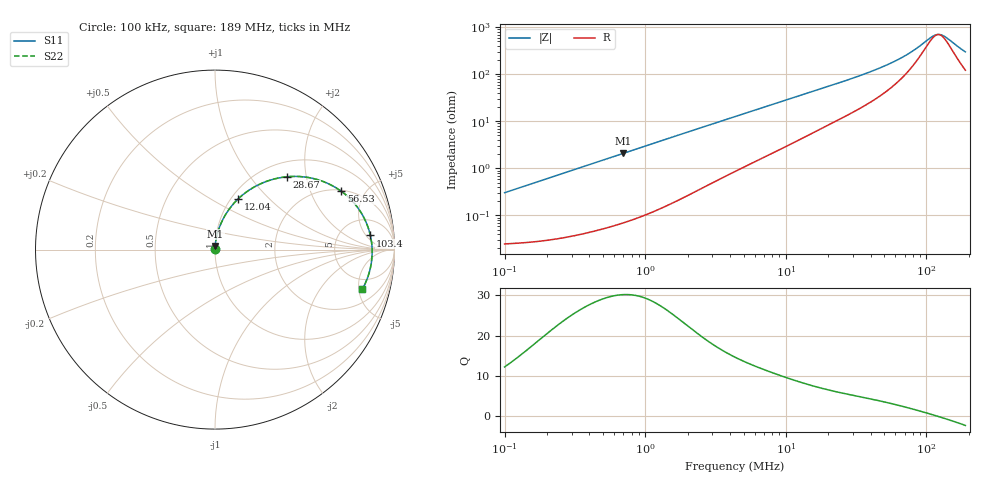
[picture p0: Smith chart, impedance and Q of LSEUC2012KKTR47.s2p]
! LSEUC2012KKTR47  S-PARAMETER MODEL  ( General Type )
! Model Generated by TAIYO YUDEN Corporation (http://www.ty-top.com)
! Version 1.0
! TAIYO YUDEN Control No. 211126
! Copyright(c) 2021 TAIYO YUDEN CO.,LTD. All Rights Reserved.
! Product Description (link to TY-COMPAS)
! https://ds.yuden.co.jp/TYCOMPAS/or/detail?pn=LSEUC2012KKTR47M&u=M
! Products Name : Inductors
! Characteristics :
!  Inductance : 0.47 uH , SRF(min) : -Hz , DC Resistance(max) : 0.027 Ohm
!  Rated Current : Saturation :5000 mA , Temp Rise : 4300 mA (40 degC)
!  Case Size : 2.0 x 1.2 / 0.079 x 0.047 [mm/inch] , Thickness : 1 / 0.039 [mm/inch]
!  (Conditions: Temperature = 25 degC , DC Bias Current/Voltage = 0A / 0V)
! External Node Assignments :
!  1  o---GGG---o  2
! GND o---------o GND
! Frequency Range : 0.1MHz  -  189.042664MHz  [ 402 STEP ]
# MHz S RI R 50
! Freq[MHz].  S11 Real  S11 Imag  S21 Real  S21 Imag  S12 Real  S12 Imag  S22 Real  S22 Imag
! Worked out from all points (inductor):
!   401 points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, 100 kHz to 189 MHz, reference 50 ohm
!   read as one part in series: L = 482 nH near 103.8 kHz
!   highest Q = 30.1 at 697.8 kHz (marker M1), where L = 476 nH
!   self-resonance near 121 MHz
!   S11 on the Smith chart (normalised r, x): 100 kHz: 1.00, +0.01; 12.04 MHz: 1.08, +0.67; 28.67 MHz: 1.29, +1.56; 56.53 MHz: 2.06, +3.36; 103.4 MHz: 10, +6; 189 MHz: 3.45, -5.46
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0.1  0.000257 0.00303  0.9997 -0.00303  0.9997 -0.00303  0.000257 0.00303
0.353854  0.000513 0.0106  0.9995 -0.0106  0.9995 -0.0106  0.000513 0.0106
0.697773  0.00113 0.0208  0.9989 -0.0208  0.9989 -0.0208  0.00113 0.0208
1.252125  0.00272 0.0371  0.9973 -0.0371  0.9973 -0.0371  0.00272 0.0371
2.469096  0.00881 0.0717  0.9912 -0.0717  0.9912 -0.0717  0.00881 0.0717
4.347904  0.0237 0.1217  0.9763 -0.1217  0.9763 -0.1217  0.0237 0.1217
7.656352  0.0616 0.1995  0.9384 -0.1995  0.9384 -0.1995  0.0616 0.1995
12.0397  0.1277 0.2813  0.8723 -0.2813  0.8723 -0.2813  0.1277 0.2813
15.38522  0.1842 0.3274  0.8158 -0.3274  0.8158 -0.3274  0.1842 0.3274
20.80492  0.2772 0.3764  0.7228 -0.3764  0.7228 -0.3764  0.2772 0.3764
28.66948  0.4027 0.4059  0.5973 -0.4059  0.5973 -0.4059  0.4027 0.4059
39.50697  0.5462 0.3964  0.4538 -0.3964  0.4538 -0.3964  0.5462 0.3964
54.44117  0.688 0.3358  0.312 -0.3358  0.312 -0.3358  0.688 0.3358
56.53407  0.7033 0.3252  0.2967 -0.3252  0.2967 -0.3252  0.7033 0.3252
76.44915  0.8068 0.2172  0.1932 -0.2172  0.1932 -0.2172  0.8068 0.2172
87.23936  0.8387 0.1593  0.1613 -0.1593  0.1613 -0.1593  0.8387 0.1593
103.3796  0.8656 0.0787  0.1344 -0.0787  0.1344 -0.0787  0.8656 0.0787
115.7666  0.8741 0.0225  0.1259 -0.0225  0.1259 -0.0225  0.8741 0.0225
127.2156  0.8753 -0.0252  0.1247 0.0252  0.1247 0.0252  0.8753 -0.0252
137.1848  0.8724 -0.0634  0.1276 0.0634  0.1276 0.0634  0.8724 -0.0634
172.0295  0.8425 -0.1758  0.1575 0.1758  0.1575 0.1758  0.8425 -0.1758
189.0427  0.8207 -0.2202  0.1793 0.2202  0.1793 0.2202  0.8207 -0.2202
